FUNCTION_BLOCK FB_AddAllAxes  //将轴添加进轴组
VAR_INPUT
	Execute				: BOOL;
END_VAR
VAR_OUTPUT
	Done				: BOOL;
	Busy				: BOOL;
	Error				: BOOL;
END_VAR
VAR
	fbAddAxis			: ARRAY[1..4] OF MC_AddAxisToGroup;
	i					: UINT;
END_VAR

Done := TRUE;
Busy := FALSE;
Error := FALSE;

fbAddAxis[1].IdentInGroup := MCS_X; //X-Axis
fbAddAxis[2].IdentInGroup := MCS_Y; //Y-Axis
fbAddAxis[3].IdentInGroup := MCS_Z; //Z-Axis
fbAddAxis[4].IdentInGroup := MCS_C1;//1st rotation is C-rotation (around Z-Axis)


fbAddAxis[1](AxesGroup:=stGroupRef, Axis := AxisArray[5], Execute := Execute);
fbAddAxis[2](AxesGroup:=stGroupRef, Axis := AxisArray[6], Execute := Execute);
fbAddAxis[3](AxesGroup:=stGroupRef, Axis := AxisArray[7], Execute := Execute);
fbAddAxis[4](AxesGroup:=stGroupRef, Axis := AxisArray[4], Execute := Execute);


FOR i:=1 TO 4 DO
	IF (NOT fbAddAxis[i].Done) THEN
		Done := FALSE;
	END_IF
	IF (fbAddAxis[i].Busy) THEN
		Busy := TRUE;
	END_IF
	IF (fbAddAxis[i].Error) THEN
		Error := TRUE;
	END_IF
END_FOR

END_FUNCTION_BLOCK
